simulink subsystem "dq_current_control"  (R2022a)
settings: Solver=VariableStepAuto  StartTime=0.0  StopTime=10.0  RelTol=1e-3
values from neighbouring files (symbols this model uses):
  Vg_ff = Vgpk    (= 21.5)    [inverter_control_params_FR.m]

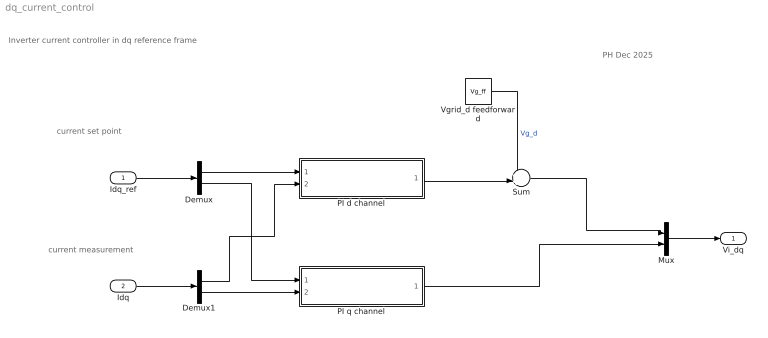
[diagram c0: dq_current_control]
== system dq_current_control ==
  note: Inverter current controller in dq reference frame
  note: current set point
  note: current measurement
  note: PH Dec 2025
  Idq_ref : Inport
  Idq : Inport  Port=2
  Demux : Demux  Outputs=2
  Demux1 : Demux  Outputs=2
  Mux : Mux  Inputs=2
  PI d channel : Subsystem  ReferencedSubsystem=pi_current
  PI q channel : Subsystem  ReferencedSubsystem=pi_current
  Sum : Sum  Inputs=++|
  Vgrid_d feedforward : Constant  Value=Vg_ff
  Vi_dq : Outport
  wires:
  Idq_ref/1 -> Demux/1
  Mux/1 -> Vi_dq/1
  Idq/1 -> Demux1/1
  Vgrid_d feedforward/1 -> Sum/1  "Vg_d"
  Sum/1 -> Mux/1
  Demux/1 -> PI d channel/1
  Demux/2 -> PI q channel/1
  Demux1/1 -> PI d channel/2
  Demux1/2 -> PI q channel/2
  PI d channel/1 -> Sum/2
  PI q channel/1 -> Mux/2
